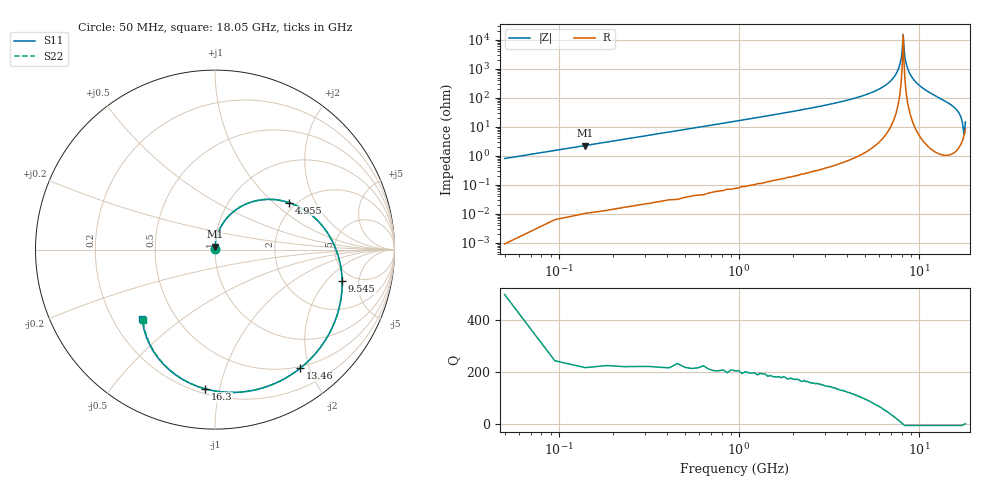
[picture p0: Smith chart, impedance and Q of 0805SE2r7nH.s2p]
! AVX Thin Film Operation		Date: May 2002
! Description: Accu-L® Series, Thin Film, SMD, RF Inductors
! Part Number: L08052R7CEWTR
! 50 MHz  -  18.05 GHz
! Serial Measurements
# mhz S db R 50
!	S11		S21		S12		S22
!	dB	Phase	dB	Phase	dB	Phase	dB	Phase
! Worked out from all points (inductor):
!   401 points, 50 MHz to 18.05 GHz, reference 50 ohm
!   read as 1/Y11, port 2 shorted: L = 2.56 nH near 140 MHz
!   highest Q = 226 at 140 MHz (marker M1), where L = 2.57 nH
!   self-resonance near 8.105 GHz
!   S11 on the Smith chart (normalised r, x): 50 MHz: 1.00, +0.01; 4.955 GHz: 1.84, +1.26; 9.545 GHz: 4.02, -3.04; 13.46 GHz: 0.47, -1.85; 16.3 GHz: 0.23, -0.90; 18.05 GHz: 0.32, -0.36
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50  -44.97 89.1  -0.00 -0.6  -0.00 -0.6  -44.97 89.1
140  -36.03 88.0  -0.00 -1.7  -0.00 -1.7  -36.03 88.0
230  -31.72 86.9  -0.00 -2.8  -0.00 -2.8  -31.72 86.9
410  -26.70 84.7  -0.01 -4.9  -0.01 -4.9  -26.70 84.7
635  -22.91 82.0  -0.03 -7.6  -0.03 -7.6  -22.91 82.0
905  -19.86 78.8  -0.05 -10.8  -0.05 -10.8  -19.86 78.8
1265  -16.99 74.5  -0.10 -15.1  -0.10 -15.1  -16.99 74.4
1760  -14.20 68.6  -0.18 -21.0  -0.18 -21.0  -14.20 68.6
3065  -9.71 53.4  -0.52 -36.2  -0.52 -36.2  -9.71 53.4
4955  -6.23 32.4  -1.23 -57.1  -1.23 -57.1  -6.23 32.4
6080  -4.95 20.6  -1.73 -68.9  -1.73 -68.9  -4.95 20.5
7610  -3.73 5.1  -2.47 -84.4  -2.47 -84.4  -3.73 5.0
9050  -2.95 -9.1  -3.18 -98.6  -3.18 -98.6  -2.95 -9.2
9545  -2.73 -14.0  -3.42 -103.5  -3.42 -103.5  -2.73 -14.1
10805  -2.30 -26.4  -4.01 -115.9  -4.01 -115.9  -2.30 -26.5
12065  -1.99 -39.2  -4.54 -128.7  -4.54 -128.7  -1.99 -39.2
13460  -1.79 -54.3  -4.98 -144.1  -4.98 -144.1  -1.79 -54.3
15080  -1.80 -74.7  -5.11 -165.0  -5.11 -165.0  -1.80 -74.6
16295  -2.19 -94.2  -4.66 174.6  -4.66 174.6  -2.18 -93.9
17150  -2.96 -112.0  -3.86 155.3  -3.86 155.3  -2.96 -111.6
17600  -3.75 -123.4  -3.26 142.6  -3.26 142.6  -3.74 -122.9
18050  -5.05 -136.5  -2.59 127.5  -2.59 127.5  -5.04 -135.9
